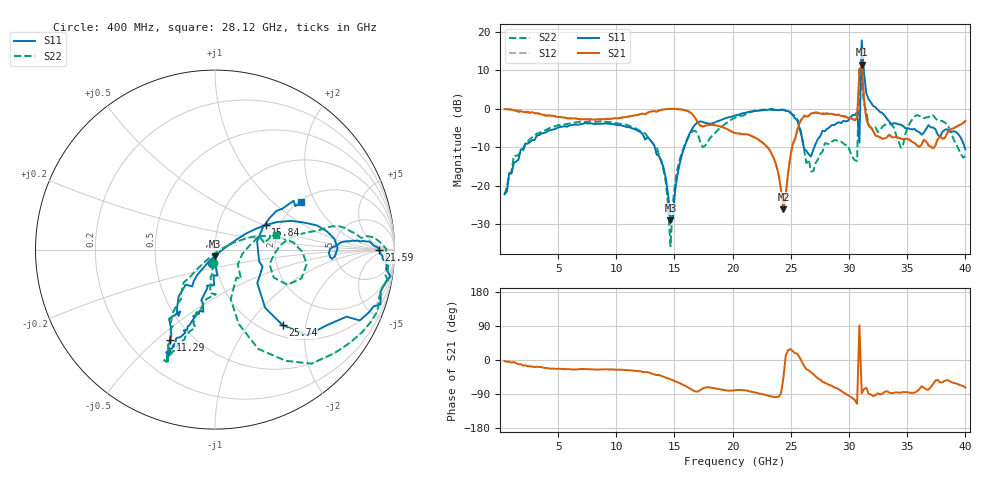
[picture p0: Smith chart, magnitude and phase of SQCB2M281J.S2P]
! Network Analyzer HP8722ES.07.66: Jul 25, 2000 Serial No. US39175408
! 27 Oct 2004  14:10:46
! Frequency  S11  S21  S12  S22
# HZ  S  DB R  50
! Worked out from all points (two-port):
!   201 points, 400 MHz to 40 GHz, reference 50 ohm
!   highest |S21| = 11.38 dB at 31.09 GHz (marker M1); lowest = -26.1 dB at 24.36 GHz (marker M2)
!   |S21| within 3 dB of the highest: 30.87 GHz to 31.16 GHz (289.9 MHz wide, 0.935 % of centre)
!   lowest |S11| = -29.0 dB at 14.66 GHz (marker M3), VSWR 1.07, Z = 49.9 - j3.52 ohm
!   |S11| at or under -10 dB: start of sweep to 2.048 GHz; 13.3 GHz to 15.85 GHz (2.548 GHz wide, 17.5 % of centre); 26.11 GHz to 27.02 GHz (903.6 MHz wide, 3.4 % of centre)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
!   |S22| runs from -35.7 to 10.3 dB; largest |S21 - S12| = 1.1
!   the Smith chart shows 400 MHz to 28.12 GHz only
!   S11 on the Smith chart (normalised r, x): 400 MHz: 0.96, -0.15; 11.29 GHz: 0.38, -0.55; 15.84 GHz: 1.69, +0.51; 21.59 GHz: 22, -1; 25.74 GHz: 1.20, -1.49; 28.12 GHz: 2.06, +1.55
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4e8  -22.21 -101.5  -0.14 -2.9  -0.11 -2.5  -22.41 -99.2
2.578e9  -8.71 -104.0  -1.05 -16.7  -1.19 -16.0  -7.86 -105.9
7.132e9  -3.96 -113.7  -2.79 -23.7  -2.89 -24.7  -3.52 -113.5
1.129e10  -5.04 -116.5  -1.95 -27.4  -1.95 -27.7  -4.68 -116.2
1.3666e10  -12.35 -121.9  -0.52 -39.6  -0.47 -39.8  -11.97 -133.6
1.4656e10  -29.05 -90.3  -0.12 -50.9  -0.07 -51.4  -35.71 -51.9
1.5052e10  -21.42 19.4  -0.06 -55.7  -0.09 -56.1  -19.32 20.4
1.5844e10  -10.06 25.9  -0.40 -66.8  -0.34 -67.1  -9.61 13.2
2.02e10  -1.82 3.2  -6.32 -79.9  -6.33 -79.5  -2.39 7.8
2.1586e10  -0.79 -0.2  -7.09 -83.7  -7.03 -83.9  -0.82 3.2
2.4358e10  -0.26 -18.3  -26.11 -48.1  -26.34 -45.1  -0.38 -24.7
2.5744e10  -4.95 -48.1  -3.79 7.4  -3.45 6.1  -4.39 -66.5
2.6932e10  -10.62 24.9  -1.14 -37.6  -1.23 -39.0  -16.23 -9.1
2.812e10  -5.22 28.7  -1.37 -63.0  -1.11 -63.8  -9.10 13.2
3.0694e10  -0.92 2.0  -2.30 -115.6  -2.25 -114.4  -13.58 94.3
3.0892e10  -8.83 -165.8  9.89 91.6  6.79 78.2  10.31 -5.4
3.109e10  17.69 -38.1  11.38 -87.8  11.10 -88.2  6.72 -125.7
3.1288e10  9.17 -47.3  2.55 -76.6  2.42 -76.5  1.35 -81.0
3.1486e10  3.96 -43.8  -2.75 -73.3  -2.79 -74.5  -0.71 -65.3
3.3466e10  -3.44 -118.1  -6.84 -86.0  -6.75 -85.6  -4.00 -152.9
3.703e10  -4.87 132.2  -9.89 -71.5  -9.83 -71.0  -1.63 134.6
4e10  -10.59 18.2  -3.19 -72.7  -3.16 -71.7  -12.34 35.6
